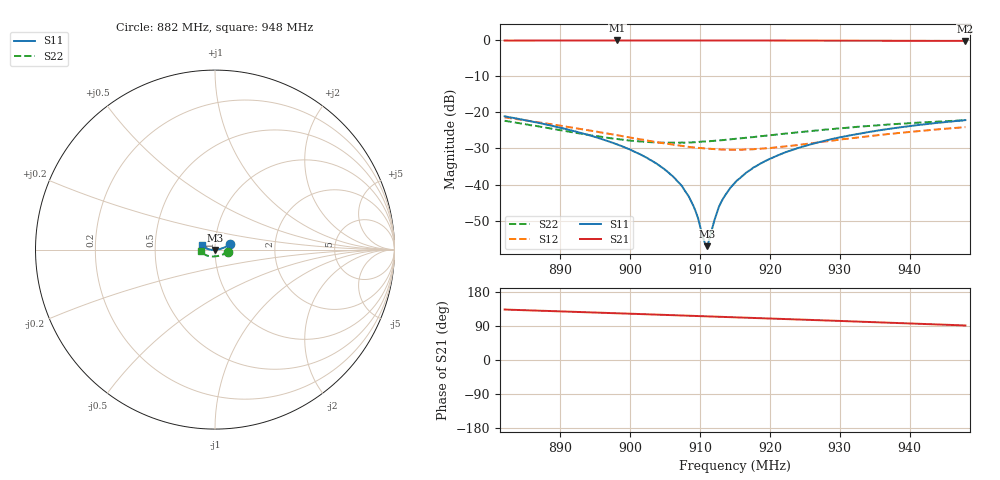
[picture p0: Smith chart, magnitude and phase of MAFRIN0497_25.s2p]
!Part Number:  MAFRIN0497
!Name:  MariaCraven
!Comments:  1
!Thu 30/Sep/2004 12:23:52 PM
!Temperature:  25
# MHZ  S  DB  R  50
!Freq  S11(dB)  S11(ang)  S21(dB)  S21(ang)  S12(dB)  S12(ang)  S22(dB)  S22(ang)
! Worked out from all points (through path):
!   201 points, 882 MHz to 948 MHz, reference 50 ohm
!   highest |S21| = -0.17 dB at 898.2 MHz (marker M1); lowest = -0.3 dB at 948 MHz (marker M2)
!   group delay of S21, straight-line fit = 1.77 ns
!   lowest |S11| = -57.0 dB at 911 MHz (marker M3), VSWR 1.00, Z = 50 - j0.134 ohm
!   |S11| at or under -10 dB: start of sweep to end of sweep
!   |S22| runs from -28.4 to -22.2 dB; largest |S21 - S12| = 0.98
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882  -21.14 19.0  -0.20 133.2  -21.44 102.2  -22.37 -8.9
893.22  -25.90 12.4  -0.18 126.3  -24.74 105.4  -26.03 -34.7
898.17  -28.93 8.9  -0.17 123.3  -26.38 110.0  -27.45 -51.3
901.47  -31.69 6.4  -0.18 121.2  -27.52 114.8  -28.09 -64.3
904.11  -34.69 4.2  -0.18 119.6  -28.40 119.8  -28.39 -75.2
906.42  -38.35 0.7  -0.17 118.1  -29.05 125.1  -28.43 -85.1
907.41  -40.43 -2.3  -0.18 117.5  -29.32 127.8  -28.41 -89.3
908.4  -43.37 -6.5  -0.18 116.9  -29.59 130.5  -28.35 -93.0
909.06  -45.99 -11.1  -0.18 116.5  -29.75 132.5  -28.31 -95.7
909.72  -49.38 -19.9  -0.18 116.1  -29.86 134.4  -28.25 -98.2
910.71  -56.36 -71.9  -0.18 115.4  -30.04 137.5  -28.09 -101.9
911.04  -57.03 -108.0  -0.18 115.2  -30.08 138.5  -28.06 -103.1
912.03  -50.00 -154.3  -0.18 114.6  -30.20 141.7  -27.89 -106.4
912.69  -46.17 -163.3  -0.18 114.2  -30.29 144.0  -27.80 -108.7
913.68  -42.72 -167.7  -0.19 113.6  -30.39 147.1  -27.62 -111.9
915  -39.46 -171.8  -0.19 112.7  -30.36 151.6  -27.41 -116.3
916.65  -36.65 -174.4  -0.20 111.7  -30.29 157.1  -27.06 -121.1
919.29  -33.53 -177.6  -0.20 110.0  -29.98 165.1  -26.52 -128.1
922.26  -31.04 179.8  -0.20 108.0  -29.45 172.6  -25.92 -135.0
926.22  -28.68 176.4  -0.21 105.5  -28.52 -179.6  -25.16 -142.7
937.11  -24.59 168.4  -0.25 98.4  -26.01 -168.6  -23.39 -159.7
948  -22.19 160.2  -0.29 91.1  -24.13 -165.2  -22.23 -173.6
